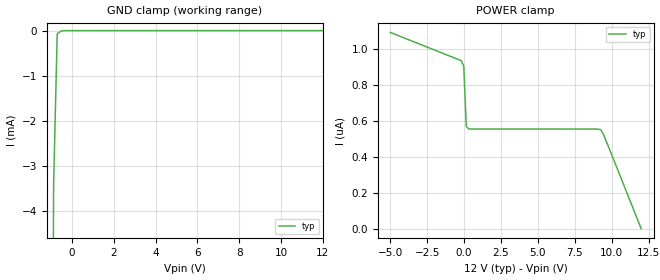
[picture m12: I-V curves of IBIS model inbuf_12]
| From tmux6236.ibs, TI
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| inbuf_12
[Model]   inbuf_12
Model_type   Input
Vinl = 0.8
Vinh = 1.3
|   typ   min   max
C_comp   4.014581e-13   NA   NA
[Voltage Range]   12   NA   NA
[Temperature Range]   27   NA   NA
[Power Clamp Reference]   12   NA   NA
[GND Clamp Reference]   0   NA   NA
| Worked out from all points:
|   GND clamp passes 1 mA (typ) near -0.75 V on its own axis
[GND Clamp]
|   Voltage   I(typ)   I(min)   I(max)
-5V       -1.213A    NA         NA
-1.051V   -21.74mA   NA         NA
-878.8mV  -3.404mA   NA         NA
-707.1mV  -74.9uA    NA         NA
-535.4mV  -10.85uA   NA         NA
12V       884.6nA    NA         NA
[POWER Clamp]
|   Voltage   I(typ)   I(min)   I(max)
-5V       1.095uA    NA         NA
-191.9mV  937.6nA    NA         NA
-20.2mV   907.1nA    NA         NA
151.5mV   570.4nA    NA         NA
323.2mV   556.2nA    NA         NA
8.737V    555.9nA    NA         NA
9.253V    551.7nA    NA         NA
9.424V    529.1nA    NA         NA
9.596V    495.3nA    NA         NA
12V       -74.97pA   NA         NA
